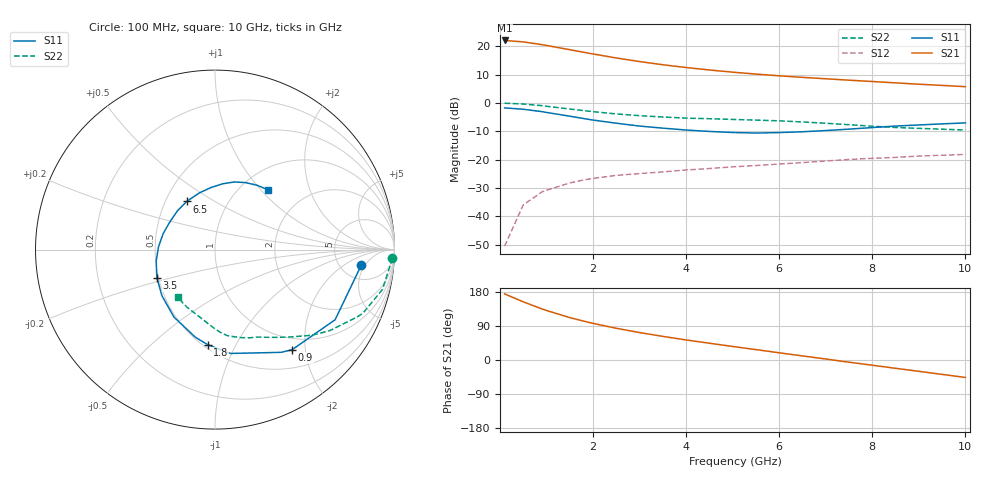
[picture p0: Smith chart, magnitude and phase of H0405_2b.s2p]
!HBFP-0405
!S-PARAMETERS at Vce=2V  Ic=5mA.  LAST UPDATED 05-29-98
# ghz s ma r 50
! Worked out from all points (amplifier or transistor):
!   23 points, 100 MHz to 10 GHz, reference 50 ohm
!   highest |S21| = 22.0 dB at 100 MHz (marker M1)
!   |S21| within 3 dB of that: start of sweep to 1.416 GHz
!   unconditionally stable (mu >= 1): 3.302 GHz to end of sweep
!   at 1 GHz: K = 0.27, MSG = 25.5 dB, |S12| = -30.8 dB
!   at 4.5 GHz: K = 1.22, MAG = 14.5 dB, |S12| = -23.1 dB
!   at 10 GHz: K = 1.45, MAG = 7.9 dB, |S12| = -18.1 dB
!   lowest NFmin = 1.36 dB at 900 MHz
!   S11 on the Smith chart (normalised r, x): 100 MHz: 7.78, -4.18; 900 MHz: 0.79, -1.75; 1.8 GHz: 0.53, -0.78; 3.5 GHz: 0.49, -0.18; 6.5 GHz: 0.64, +0.38; 10 GHz: 1.33, +1.10
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0.1  0.819 -6.2  12.63 174.5  0.003 87.8  0.99 -2.8
0.5  0.775 -30.3  11.91 153.5  0.016 77.1  0.959 -13.4
0.9  0.704 -52.4  10.66 134.9  0.027 67.3  0.897 -23.3
1  0.681 -57.2  10.31 130.7  0.029 64.9  0.875 -25.5
1.5  0.585 -81.5  8.689 111.9  0.039 54.0  0.783 -35.2
1.8  0.531 -94.5  7.817 102.5  0.044 49.0  0.733 -40.1
2  0.5 -102.7  7.306 96.7  0.047 46.0  0.703 -43.0
2.5  0.44 -121.3  6.208 83.7  0.053 39.9  0.641 -49.4
3  0.392 -138.9  5.362 72.4  0.057 34.6  0.597 -55.0
3.5  0.36 -154.1  4.716 62.3  0.061 30.4  0.566 -59.7
4  0.334 -168.9  4.214 52.9  0.066 26.5  0.541 -64.2
4.5  0.315 177.0  3.814 44.3  0.07 23.0  0.528 -68.6
5  0.302 162.5  3.491 35.7  0.075 19.0  0.513 -73.0
5.5  0.295 148.1  3.229 27.4  0.079 15.1  0.499 -77.0
6  0.301 133.7  3.01 19.0  0.084 11.1  0.484 -82.0
6.5  0.311 120.4  2.827 10.8  0.089 6.4  0.463 -86.1
7  0.327 105.9  2.668 2.6  0.095 2.1  0.439 -90.5
7.5  0.346 94.0  2.52 -5.8  0.101 -3.0  0.414 -95.4
8  0.369 83.4  2.389 -13.8  0.106 -7.7  0.389 -101.6
8.5  0.392 74.1  2.261 -21.9  0.11 -12.8  0.37 -108.5
9.5  0.428 56.9  2.038 -38.0  0.12 -23.1  0.345 -122.3
10  0.446 48.2  1.937 -46.0  0.124 -28.5  0.334 -127.9
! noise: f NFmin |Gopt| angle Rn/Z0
0.9  1.36  0.386  2.8  0.34
1.5  1.46  0.333  17.7  0.32
2  1.55  0.292  31.9  0.31
3  1.73  0.208  59.9  0.26
4  1.93  0.153  85.6  0.24
5.5  2.18  0.065  141.5  0.24
6.5  2.37  0.068  -129.9  0.27
7.5  2.56  0.133  -82.9  0.34
8.5  2.85  0.212  -62.8  0.46
10  3.12  0.314  -37.3  0.7
